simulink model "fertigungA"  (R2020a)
settings: Solver=FixedStepDiscrete  StartTime=0.0  StopTime=25.1  RelTol=1e-3  EnableMultiTasking=on

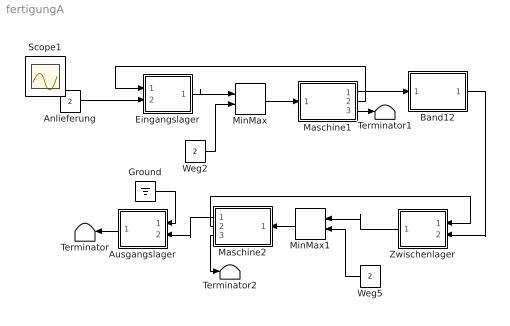
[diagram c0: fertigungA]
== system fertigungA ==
  Anlieferung : Constant  Value=2
  Ausgangslager : Subsystem  mask{m0=0, dt=1, t0=0.1}
      mask prompts: m0 "Initial Value"; dt "Sample Period"; t0 "Start Time"
  Band12 : Subsystem  mask{ndelay=3, dt=1, t0=0.1}
      mask prompts: ndelay "Transit time"; dt "Sample Period"; t0 "Start Time"
  Eingangslager : Subsystem  mask{m0=7, dt=1, t0=0.1}
      mask prompts: m0 "Initial Value"; dt "Sample Period"; t0 "Start Time"
  Ground : Ground
  Maschine1 : Subsystem  mask(Oven){cookingtime=2, capacity=4, initload=0, dt=1, t0=0.1}
      mask prompts: cookingtime "Cooking time"; initload "Initial load"; dt "Sample Period"; t0 "Start Time"
  Maschine2 : Subsystem  mask(Oven){cookingtime=1, capacity=2, initload=0, dt=1, t0=0.1}
      mask prompts: cookingtime "Cooking time"; initload "Initial load"; dt "Sample Period"; t0 "Start Time"
  MinMax : MinMax  Inputs=2  InputSameDT=on  SaturateOnIntegerOverflow=on
  MinMax1 : MinMax  Inputs=2  InputSameDT=on  SaturateOnIntegerOverflow=on
  Terminator : Terminator
  Terminator1 : Terminator
  Terminator2 : Terminator
  Weg2 : Constant  Value=2
  Weg5 : Constant  Value=2
  Zwischenlager : Subsystem  mask{m0=0, dt=1, t0=0.1}
      mask prompts: m0 "Initial Value"; dt "Sample Period"; t0 "Start Time"
  Scope1 : Scope
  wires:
  Anlieferung/1 -> Eingangslager/2(In2)
  MinMax/1 -> Maschine1/1(in)
  Eingangslager/1(Out1) -> MinMax/1
  Weg2/1 -> MinMax/2
  Maschine1/1(out) -> Band12/1(In)
  MinMax1/1 -> Maschine2/1(in)
  Weg5/1 -> MinMax1/2
  Maschine2/1(out) -> Ausgangslager/2(In2)
  Maschine1/2(increment) -> Eingangslager/1(In1)
  Ausgangslager/1(Out1) -> Terminator/1
  Maschine1/3(load) -> Terminator1/1
  Zwischenlager/1(Out1) -> MinMax1/1
  Band12/1(Out) -> Zwischenlager/2(In2)
  Maschine2/2(increment) -> Zwischenlager/1(In1)
  Maschine2/3(load) -> Terminator2/1
  Ground/1 -> Ausgangslager/1(In1)

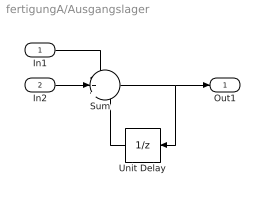
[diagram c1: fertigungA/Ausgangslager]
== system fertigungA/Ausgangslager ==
  In1 : Inport
  In2 : Inport  Port=2
  Sum : Sum  Inputs=-++  SaturateOnIntegerOverflow=on
  Unit Delay : UnitDelay  InitialCondition=m0  SampleTime=[dt, t0]  HasFrameUpgradeWarning=on
  Out1 : Outport
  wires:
  Unit Delay/1 -> Sum/3
  In2/1 -> Sum/2
  Sum/1 -> Unit Delay/1, Out1/1
  In1/1 -> Sum/1

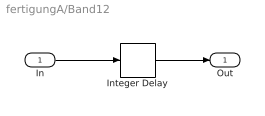
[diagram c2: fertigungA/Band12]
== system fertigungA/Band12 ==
  In : Inport
  Integer Delay : Delay  DelayLength=ndelay  SampleTime=[dt,t0]
  Out : Outport
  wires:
  Integer Delay/1 -> Out/1
  In/1 -> Integer Delay/1

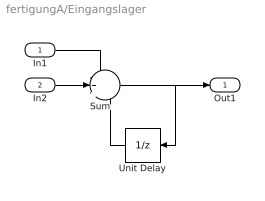
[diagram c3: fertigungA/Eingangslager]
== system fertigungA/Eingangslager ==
  In1 : Inport
  In2 : Inport  Port=2
  Sum : Sum  Inputs=-++  SaturateOnIntegerOverflow=on
  Unit Delay : UnitDelay  InitialCondition=m0  SampleTime=[dt, t0]  HasFrameUpgradeWarning=on
  Out1 : Outport
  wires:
  Unit Delay/1 -> Sum/3
  In2/1 -> Sum/2
  Sum/1 -> Unit Delay/1, Out1/1
  In1/1 -> Sum/1

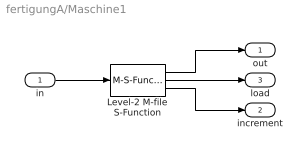
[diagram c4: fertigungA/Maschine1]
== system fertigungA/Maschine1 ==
  in : Inport
  Level-2 M-file S-Function : M-S-Function  FunctionName=sfun_oven  Parameters=capacity, cookingtime, initload, dt, t0
  out : Outport
  increment : Outport  Port=2
  load : Outport  Port=3
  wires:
  Level-2 M-file S-Function/3 -> increment/1
  Level-2 M-file S-Function/2 -> load/1
  Level-2 M-file S-Function/1 -> out/1
  in/1 -> Level-2 M-file S-Function/1

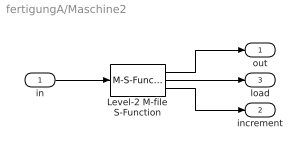
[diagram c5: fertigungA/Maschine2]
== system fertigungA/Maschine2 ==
  in : Inport
  Level-2 M-file S-Function : M-S-Function  FunctionName=sfun_oven  Parameters=capacity, cookingtime, initload, dt, t0
  out : Outport
  increment : Outport  Port=2
  load : Outport  Port=3
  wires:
  Level-2 M-file S-Function/3 -> increment/1
  Level-2 M-file S-Function/2 -> load/1
  Level-2 M-file S-Function/1 -> out/1
  in/1 -> Level-2 M-file S-Function/1

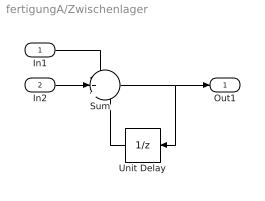
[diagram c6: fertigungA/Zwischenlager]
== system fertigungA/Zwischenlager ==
  In1 : Inport
  In2 : Inport  Port=2
  Sum : Sum  Inputs=-++  SaturateOnIntegerOverflow=on
  Unit Delay : UnitDelay  InitialCondition=m0  SampleTime=[dt, t0]  HasFrameUpgradeWarning=on
  Out1 : Outport
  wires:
  Unit Delay/1 -> Sum/3
  In2/1 -> Sum/2
  Sum/1 -> Unit Delay/1, Out1/1
  In1/1 -> Sum/1
